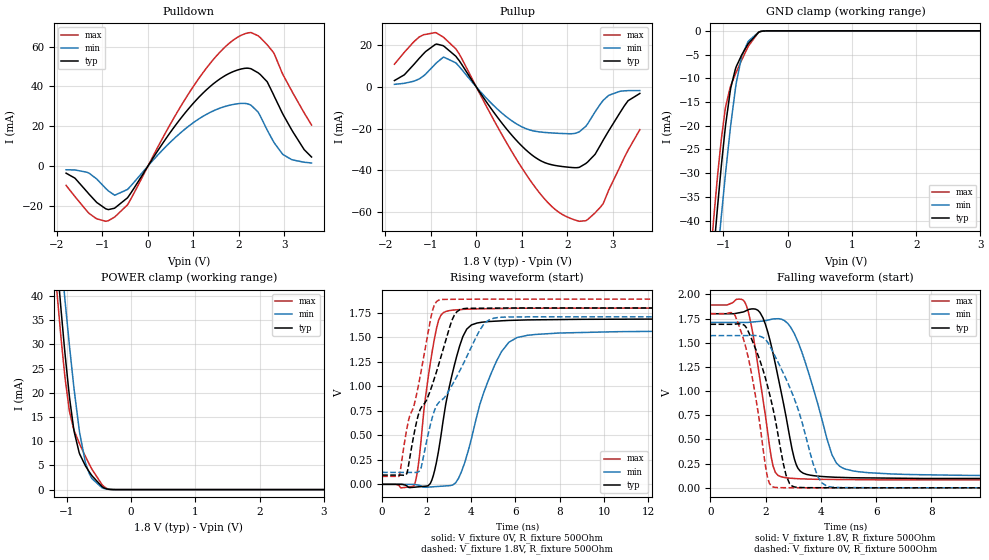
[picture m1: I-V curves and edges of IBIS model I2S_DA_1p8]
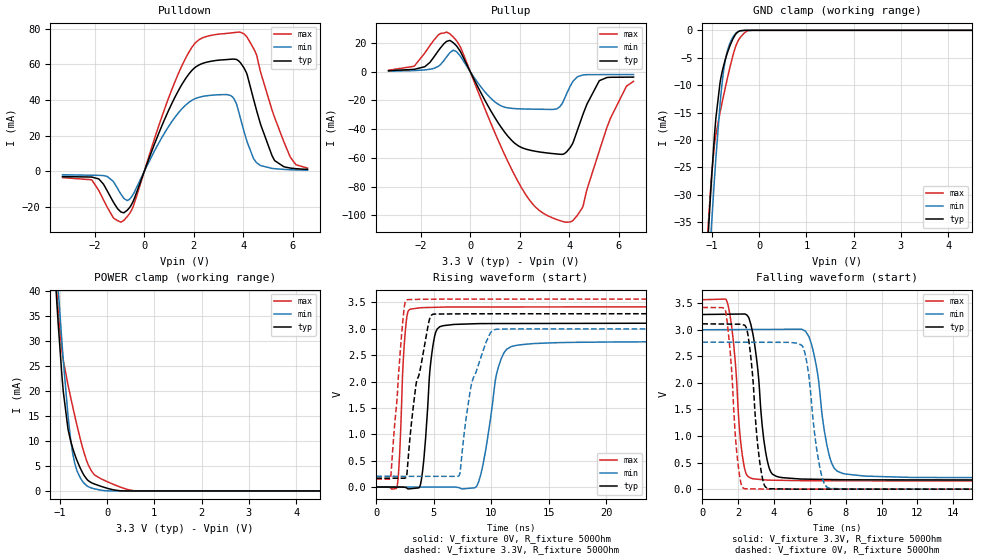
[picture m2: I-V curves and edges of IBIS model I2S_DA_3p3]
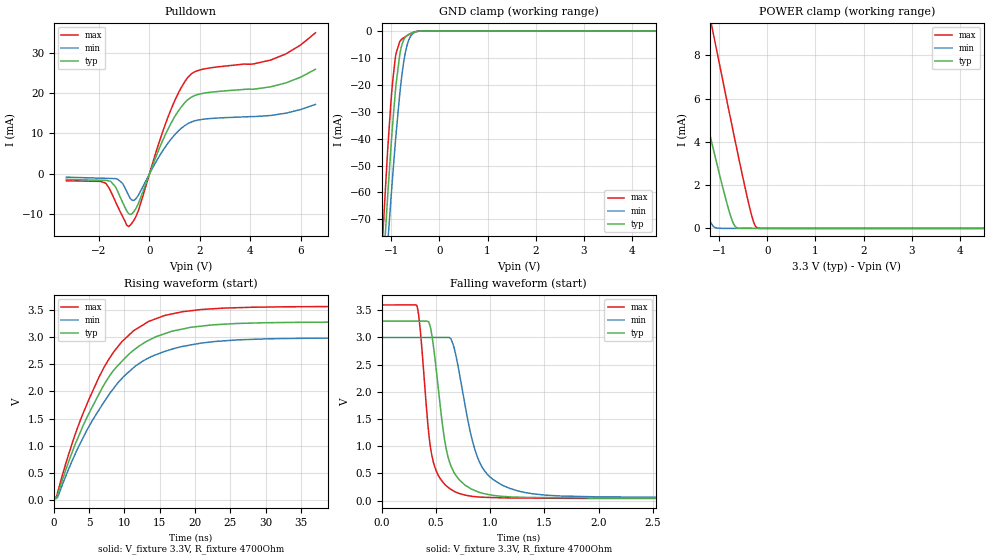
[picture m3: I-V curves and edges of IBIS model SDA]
| Texas Instruments Incorporated
| DS90UH928Q
| 5-85MHz 24-bit Color FPD-Link III to FPD-Link Deserializer with HDCP
| Marketing part#   Voltage Range   Package-type   Temperature
| DS90UH928QSQE   1.71V - 3.6V   48-Pin LLP   -40 to 105C
| DS90UH928QSQ   1.71V - 3.6V   48-Pin LLP   -40 to 105C
| DS90UH928QSQX   1.71V - 3.6V   48-Pin LLP   -40 to 105C
[IBIS Ver]   4.1
[File name]   ds90uh928q.ibs
[File Rev]   1.1
[Date]   08/10/2015
[Source]   Model built from SPICE simulations at:
   Texas Instruments Incorporated.
   WEBENCH DESIGN CENTER
   12500 TI Blvd
   Dallas, TX -75243
[Notes]   Rev 1.1: 08/10/2015
   - Diff pin mapping corrected.
   Rev 1.0: 02/13/2013
   - Initial version of the IBIS model
   - All models are generated in Spectre
   - ccomp is listed in numerical order, for PVT information,
   please check notes above ccomp keyword for each model
   - All non-monotonic warnings can be ignored as they were reviewed and
   considered minor.
   - Models with trailing xxxx_1p8 and xxxx_3p3 represent 1.8V and 3.3V
   power supply operation respectively.
[Disclaimer] This product is designed as an aid for customers of Texas Instruments.
   No warranties, either expressed or implied, with respect to this third
   party software (if any) or with respect to its fitness for any
   particular purpose is claimed by Texas Instruments or the author. The
   software (if any) is provided solely on an "as is" basis. The entire
   risk as to its quality and performance is with the customer
[Copyright]   (C)Copyright 2013 Texas Instruments Incorporated.
   All rights reserved.
[Component]   DS90UH928Q
[Manufacturer]  Texas Instruments, Inc.
[Package]   |48-pin LLP
|   typ   min   max
R_pkg   0   0   0
L_pkg   0   0   0
C_pkg   0   0   0
[Pin]   signal_name   model_name   R_pin   L_pin   C_pin
1   PDB   PDB
2   CAPI2S   NC
3   I2S_DB/GPIO_REG5   I2S_DA
4   SDA   SDA
5   SCL   SDA
6   VDDIO   POWER
7   I2S_DA/GPIO_REG6   I2S_DA
8   I2S_CLK/GPIO_REG8   I2S_DA
9   BISTTEN   OEN
10   I2S_WC/GPIO_REG7   I2S_DA
11   MCLK   I2S_DA
12   IDX   NC
13   GPIO1   I2S_DA
14   GPIO0   I2S_DA
15   TXOUT3+   LVDS_OUT
16   TXOUT3-   LVDS_OUT
17   TXCLKOUT+   LVDS_OUT
18   TXCLKOUT-   LVDS_OUT
19   TXOUT2+   LVDS_OUT
20   TXOUT2-   LVDS_OUT
21   TXOUT1+   LVDS_OUT
22   TXOUT1-   LVDS_OUT
23   TXOUT0+   LVDS_OUT
24   TXOUT0-   LVDS_OUT
25   CAPLV25   NC
26   MAPSEL   OEN
27   LOCK   I2S_DA
28   PASS   I2S_DA
29   CAPLV12   NC
30   OEN   OEN
31   VDD33_B   POWER
32   LFMODE   OEN
33   CAPL12   NC
34   RES0   NC
35   OSS_SEL   OEN
36   I2S_DD/GPIO3   I2S_DA
37   I2S_DC/GPIO2   I2S_DA
38   VDD33_A   POWER
39   RES1   NC
40   RIN+   RX_CML_RCV
41   RIN-   RX_CML_RCV
42   CMF   NC
43   BISTC/INTB_IN   OEN
44   CMLOUTP   RX_CML
45   CMLOUTN   RX_CML
46   CAPR12   NC
47   CAPP12   NC
48   MODE_SEL   NC
49   DAP   GND
[Package Model] LLP48DS90UH928QSQ
[Diff pin]  inv_pin  vdiff  tdelay_typ  tdelay_min  tdelay_max
17   18   NA   NA   NA   NA
15   16   NA   NA   NA   NA
19   20   NA   NA   NA   NA
21   22   NA   NA   NA   NA
23   24   NA   NA   NA   NA
40   41   0.2   NA   NA   NA
44   45   0.2   NA   NA   NA
|   Model Selectors
[Model Selector]  I2S_DA
I2S_DA_3p3   3.3V operation
I2S_DA_1p8   3.3V operation
[Model Selector]  OEN
OEN_3p3   3.3V operation
OEN_1p8   3.3V operation
[Define Package Model]  LLP48DS90UH928QSQ
[Manufacturer]  Texas Instruments
[OEM]  Texas Instruments
[Description]  None
[Number Of Pins]  49
[Pin Numbers]
|Pin Num   Terminal Name
1   | L1:1
2   | L2:2
3   | L3:3
4   | L4:4
5   | L5:5
6   | L6:6
7   | L7:7
8   | L8:8
9   | L9:9
10   | L10:10
11   | L11:11
12   | L12:12
13   | L13:13
14   | L14:14
15   | L15:15
16   | L16:16
17   | L17:17
18   | L18:18
19   | L19:19
20   | L20:20
21   | L21:21
22   | L22:22
23   | L23:23
24   | L24:24
25   | L25:25
26   | L26:26
27   | L27:27
28   | L28:28
29   | L29:29
30   | L30:30
31   | L31:31
32   | L32:32
33   | L33:33
34   | L34:34
35   | L35:35
36   | L36:36
37   | L37:37
38   | L38:38
39   | L39:39
40   | L40:40
41   | L41:41
42   | L42:42
43   | L43:43
44   | L44:44
45   | L45:45
46   | L46:46
47   | L47:47
48   | L48:48
49   | LDAP:49
[Model Data]
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[End Model Data]
[End Package Model]
| Models and submodels in the file (9): I2S_DA_1p8 (I/O), I2S_DA_3p3 (I/O), SDA (I/O_open_drain), RX_CML_RCV (Input), RX_CML (Output), PDB (Input), OEN_3p3 (Input), OEN_1p8 (Input), LVDS_OUT (Output)
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|   Model
[Model]   I2S_DA_1p8
Model_type   I/O
Polarity   Non-Inverting
Enable   Active-Low
Vinl = 0.63
Vinh = 1.17
Vmeas = 0.9
Vref = 0
Cref = 1pF
Rref = 1000000
|   typ   min   max
C_comp   1.5999pF   1.5084pF   1.9148pF
[Voltage Range]   1.8   1.71   1.89
[Temperature Range]   25   105   -40
[Pullup Reference]   1.8   1.71   1.89
[Pulldown Reference]   0   0   0
[Power Clamp Reference]   1.8   1.71   1.89
[GND Clamp Reference]   0   0   0
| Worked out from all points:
|   slope of the pulldown table from 0 to 0.27 V, typ, clamps not added: 28.2 ohm
|   slope of the pullup table from 0 to 0.27 V, typ, clamps not added: 31.1 ohm
|   GND clamp passes 1 mA (typ) near -0.50 V on its own axis
|   POWER clamp passes 1 mA (typ) near -0.48 V on its own axis
|   falling waveform, V_fixture 1.8V, R_fixture 500Ohm: 20-80 % time 720ps typ, 970ps min, 560ps max; typ from 1.8 V to 0.094 V
|   rising waveform, V_fixture 0V, R_fixture 500Ohm: 20-80 % time 877ps typ, 1.31ns min, 607ps max; typ from 0 V to 1.69 V
|   rising waveform, V_fixture 1.8V, R_fixture 500Ohm: 20-80 % time 1.48ns typ, 2ns min, 1.03ns max; typ from 0.094 V to 1.8 V
|   falling waveform, V_fixture 0V, R_fixture 500Ohm: 20-80 % time 835ps typ, 1.14ns min, 636ps max; typ from 1.69 V to 0 V
[Pulldown]
|   Voltage   I(typ)   I(min)   I(max)
-1.8V     -3.602mA   -1.89mA    -9.732mA
-1.13V    -18.2mA    -6.438mA   -26.49mA
-730.8mV  -21.14mA   -14.67mA   -25.6mA
-450mV    -15.96mA   -11.77mA   -19.49mA
457.2mV   15.8mA     11.21mA    19.63mA
1.105V    34.21mA    23.45mA    43.56mA
1.705V    45.5mA     29.98mA    59.98mA
2.196V    49.12mA    31.15mA    66.83mA
2.417V    46.85mA    27.15mA    65.43mA
2.617V    42.37mA    18.18mA    60.95mA
2.957V    26.38mA    5.999mA    46.3mA
3.595V    4.522mA    1.513mA    20.6mA
[GND Clamp]
|   Voltage   I(typ)   I(min)   I(max)
-1.8V     -162.6mA   -161mA     -166.7mA
-1.201V   -55.01mA   -64.35mA   -48.08mA
-1.152V   -46.98mA   -56.91mA   -39.96mA
-1.093V   -37.56mA   -48.01mA   -30.98mA
-1.039V   -29.54mA   -40.16mA   -23.8mA
-963mV    -19.69mA   -29.71mA   -15.92mA
-892.8mV  -12.73mA   -20.82mA   -11.89mA
-795.6mV  -7.443mA   -10.75mA   -8.613mA
-714.6mV  -5.105mA   -5.442mA   -6.162mA
-617.4mV  -2.827mA   -2.355mA   -3.43mA
-450mV    -299.1uA   -264.1uA   -281.1uA
3.595V    0A         0A         0A
[Pullup]
|   Voltage   I(typ)   I(min)   I(max)
-1.8V     3.07mA     1.252mA    10.93mA
-1.255V   13.76mA    3.863mA    24.05mA
-903.6mV  20.4mA     10.96mA    26.16mA
-714.6mV  19.65mA    14.35mA    23.79mA
-374.4mV  12.6mA     9.801mA    15.82mA
457.2mV   -14.35mA   -10.52mA   -18.8mA
1.094V    -30.36mA   -20.07mA   -42.03mA
1.667V    -37.47mA   -22.14mA   -57.64mA
2.25V     -38.72mA   -21.72mA   -64.53mA
2.785V    -25.75mA   -6.573mA   -56.24mA
3.335V    -6.631mA   -1.777mA   -30.42mA
3.595V    -3.131mA   -1.752mA   -20.54mA
[POWER Clamp]
|   Voltage   I(typ)   I(min)   I(max)
-1.8V     161.3mA    160.4mA    165mA
-1.157V   48.1mA     58.18mA    41.7mA
-1.087V   37.06mA    47.82mA    31.19mA
-1.033V   29.11mA    40.11mA    24.06mA
-957.6mV  19.26mA    29.82mA    16.3mA
-882mV    11.86mA    20.43mA    12.15mA
-795.6mV  7.282mA    11.52mA    9.335mA
-709.2mV  4.933mA    5.625mA    6.87mA
-606.6mV  2.86mA     2.271mA    4.196mA
-450mV    607.2uA    381.3uA    1.019mA
-266.4mV  7.62uA     8.999uA    8.268uA
3.595V    0A         0A         0A
[Ramp]
R_load = 500
|   typ   min   max
dV/dt_r   1.01367/8.76582e-10   0.941883/1.31022e-09   1.0806/6.06669e-10
dV/dt_f   1.02351/7.20399e-10   0.952642/9.69527e-10   1.08535/5.60273e-10
[Falling Waveform]
V_fixture = 1.8V
V_fixture_min = 1.71V
V_fixture_max = 1.89V
R_fixture = 500Ohm
C_fixture = 0F
|   Time   V(typ)   V(min)   V(max)
0s        1.8V       1.71V      1.89V
1.301ns   1.832V     1.71V      1.885V
1.791ns   1.814V     1.722V     1.127V
2.269ns   1.388V     1.746V     225.1mV
2.643ns   876.4mV    1.735V     109.2mV
3.038ns   301.6mV    1.595V     97.02mV
3.255ns   171.8mV    1.447V     93.41mV
4.404ns   111.4mV    341.2mV    87.05mV
5.171ns   104.5mV    174.8mV    85.19mV
30ns      94.14mV    122.3mV    81.06mV
[Rising Waveform]
V_fixture = 0V
V_fixture_min = 0V
V_fixture_max = 0V
R_fixture = 500Ohm
C_fixture = 0F
|   Time   V(typ)   V(min)   V(max)
0s        4.816uV    9.619uV    3.008uV
1.493ns   -28.51mV   -2.803mV   21.83mV
2.243ns   45.32mV    -25.87mV   1.338V
2.544ns   345mV      -21.27mV   1.674V
2.894ns   849.8mV    -15.93mV   1.766V
3.311ns   1.264V     14.84mV    1.78V
3.81ns    1.583V     289.4mV    1.788V
5.032ns   1.664V     1.196V     1.793V
6.083ns   1.675V     1.498V     1.797V
30ns      1.689V     1.57V      1.801V
[Rising Waveform]
V_fixture = 1.8V
V_fixture_min = 1.71V
V_fixture_max = 1.89V
R_fixture = 500Ohm
C_fixture = 0F
|   Time   V(typ)   V(min)   V(max)
0s        94.11mV    122.2mV    81.06mV
776.8ps   94.16mV    121.5mV    89.81mV
1.124ns   117.9mV    121.2mV    580.5mV
1.706ns   758.9mV    142.7mV    1.094V
2.269ns   1.022V     689.8mV    1.774V
2.544ns   1.22V      832.6mV    1.879V
3.361ns   1.759V     1.099V     1.888V
4.561ns   1.797V     1.628V     1.889V
5.171ns   1.798V     1.701V     1.889V
30ns      1.8V       1.71V      1.89V
[Falling Waveform]
|Gnd
V_fixture = 0V
V_fixture_min = 0V
V_fixture_max = 0V
R_fixture = 500Ohm
C_fixture = 0F
|   Time   V(typ)   V(min)   V(max)
0s        1.691V     1.574V     1.802V
990.8ps   1.696V     1.574V     1.71V
1.504ns   1.529V     1.576V     1.157V
2.041ns   1.083V     1.518V     145.5mV
2.269ns   814.3mV    1.402V     9.432mV
2.643ns   246mV      1.184V     1.524mV
2.867ns   42.58mV    1.042V     1.319mV
3.893ns   1.5mV      114.2mV    464.1uV
4.404ns   985.5uV    6.822mV    455.2uV
30ns      18.46uV    39.95uV    10.33uV
|   Model
[Model]   I2S_DA_3p3
Model_type   I/O
Polarity   Non-Inverting
Enable   Active-Low
Vinl = 0.8
Vinh = 2
Vmeas = 1.65
Vref = 0
Cref = 1pF
Rref = 1000000
|   typ   min   max
C_comp   1.5999pF   1.5084pF   1.9148pF
[Voltage Range]   3.3   3   3.6
[Temperature Range]   25   105   -40
[Pullup Reference]   3.3   3   3.6
[Pulldown Reference]   0   0   -0
[Power Clamp Reference]   3.3   3   3.6
[GND Clamp Reference]   0   -0   0
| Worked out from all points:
|   slope of the pulldown table from 0 to 0.495 V, typ, clamps not added: 27.2 ohm
|   slope of the pullup table from 0 to 0.495 V, typ, clamps not added: 29.4 ohm
|   GND clamp passes 1 mA (typ) near -0.52 V on its own axis
|   POWER clamp passes 1 mA (typ) near -0.15 V on its own axis
|   falling waveform, V_fixture 3.3V, R_fixture 500Ohm: 20-80 % time 547ps typ, 705ps min, 459ps max; typ from 3.29 V to 0.169 V
|   rising waveform, V_fixture 0V, R_fixture 500Ohm: 20-80 % time 631ps typ, 1.15ns min, 401ps max; typ from 0 V to 3.11 V
|   rising waveform, V_fixture 3.3V, R_fixture 500Ohm: 20-80 % time 1.31ns typ, 1.55ns min, 725ps max; typ from 0.168 V to 3.29 V
|   falling waveform, V_fixture 0V, R_fixture 500Ohm: 20-80 % time 458ps typ, 570ps min, 412ps max; typ from 3.11 V to 0 V
[Pulldown]
|   Voltage   I(typ)   I(min)   I(max)
-3.3V     -2.905mA   -1.903mA   -3.487mA
-1.845V   -4.191mA   -2.225mA   -10.53mA
-825mV    -23.24mA   -15.16mA   -27.48mA
-458.7mV  -17.06mA   -13.07mA   -20.03mA
838.2mV   29.71mA    21.98mA    35.7mA
1.818V    54.9mA     38.87mA    67.25mA
3.472V    62.85mA    42.63mA    77.57mA
3.828V    61.71mA    32.59mA    78.09mA
4.412V    40.42mA    7.131mA    68.97mA
5.254V    6.237mA    1.524mA    30.5mA
5.897V    1.863mA    934.9uA    7.885mA
6.59V     1.078mA    679uA      1.807mA
[GND Clamp]
|   Voltage   I(typ)   I(min)   I(max)
-3.3V     -460mA     -423.9mA   -501.5mA
-1.073V   -36.94mA   -45.07mA   -35.22mA
-1.063V   -35.41mA   -43.62mA   -33.84mA
-1.013V   -28.09mA   -36.56mA   -27.51mA
-1.003V   -26.71mA   -35.18mA   -26.38mA
-914.1mV  -16.06mA   -23.41mA   -19.06mA
-825mV    -9.505mA   -13.43mA   -14.97mA
-745.8mV  -6.327mA   -7.116mA   -11.73mA
-617.1mV  -2.836mA   -2.348mA   -6.773mA
-419.1mV  -144.9uA   -143.6uA   -1.548mA
-132mV    -33.32nA   -83.84nA   -493.6nA
6.59V     0A         0A         0A
[Pullup]
|   Voltage   I(typ)   I(min)   I(max)
-3.3V     733uA      422.9uA    1.047mA
-1.845V   3.487mA    1.261mA    12.89mA
-825mV    21.85mA    13.3mA     26.44mA
-379.5mV  13.39mA    10.25mA    16.46mA
1.68V     -48.01mA   -25.51mA   -68.38mA
2.64V     -55.46mA   -26.1mA    -94.48mA
3.491V    -57.32mA   -25.83mA   -103mA
3.887V    -55.85mA   -15.31mA   -104.9mA
4.531V    -30.54mA   -2.272mA   -94.57mA
5.204V    -6.337mA   -1.995mA   -55.33mA
5.669V    -3.846mA   -1.979mA   -32mA
6.59V     -3.726mA   -1.961mA   -6.65mA
[POWER Clamp]
|   Voltage   I(typ)   I(min)   I(max)
-3.3V     458.5mA    424mA      498.8mA
-1.082V   40.82mA    47.39mA    42.47mA
-1.053V   36.34mA    43.15mA    38.45mA
-1.033V   33.45mA    40.37mA    35.94mA
-924mV    19.77mA    25.99mA    26.02mA
-825mV    12.34mA    14.99mA    21.17mA
-735.9mV  8.878mA    8.069mA    17.26mA
-627mV    5.889mA    3.864mA    12.75mA
-389.4mV  1.994mA    814.3uA    5.052mA
-132mV    937.8uA    161.4uA    2.443mA
561mV     0A         0A         44.45uA
6.59V     0A         0A         0A
[Ramp]
R_load = 500
|   typ   min   max
dV/dt_r   1.86529/6.30855e-10   1.65454/1.14623e-09   2.05076/4.01389e-10
dV/dt_f   1.87026/5.43355e-10   1.67581/7.00491e-10   2.04655/4.58036e-10
[Falling Waveform]
V_fixture = 3.3V
V_fixture_min = 3V
V_fixture_max = 3.6V
R_fixture = 500Ohm
C_fixture = 0F
|   Time   V(typ)   V(min)   V(max)
0s        3.286V     2.999V     3.564V
1.413ns   3.292V     3.002V     3.492V
2.214ns   3.295V     3.003V     677.9mV
2.736ns   3.056V     3.004V     203.9mV
3.524ns   713.9mV    3.005V     173.4mV
4.134ns   240.4mV    3.006V     167.6mV
5.945ns   188mV      2.87V      157.9mV
7.071ns   181.7mV    650.4mV    157.4mV
7.806ns   177.7mV    298.9mV    157.3mV
30ns      169.2mV    206.1mV    153.4mV
[Rising Waveform]
V_fixture = 0V
V_fixture_min = 0V
V_fixture_max = 0V
R_fixture = 500Ohm
C_fixture = 0F
|   Time   V(typ)   V(min)   V(max)
0s        6.519uV    10.19uV    508.7nV
1.805ns   -114.1uV   2.453uV    4.229mV
2.427ns   -3.741mV   -213.9nV   2.689V
2.91ns    -32.89mV   -2.285uV   3.367V
3.914ns   130.3mV    -6.59uV    3.401V
4.781ns   2.454V     -10.31uV   3.406V
5.509ns   3.039V     -13.43uV   3.41V
8.796ns   3.098V     44.76mV    3.414V
11.71ns   3.1V       2.662V     3.414V
30ns      3.109V     2.758V     3.418V
[Rising Waveform]
V_fixture = 3.3V
V_fixture_min = 3V
V_fixture_max = 3.6V
R_fixture = 500Ohm
C_fixture = 0F
|   Time   V(typ)   V(min)   V(max)
0s        168.4mV    203.6mV    153mV
1.255ns   167.9mV    203.4mV    175.4mV
2.225ns   167.6mV    203.3mV    2.955V
2.605ns   190.7mV    203.3mV    3.545V
3.47ns    1.968V     203.2mV    3.558V
4.902ns   3.275V     203.1mV    3.562V
7.209ns   3.283V     222.6mV    3.563V
8.285ns   3.285V     1.973V     3.563V
10.13ns   3.285V     2.968V     3.563V
30ns      3.286V     2.999V     3.564V
[Falling Waveform]
|Gnd
V_fixture = 0V
V_fixture_min = 0V
V_fixture_max = 0V
R_fixture = 500Ohm
C_fixture = 0F
|   Time   V(typ)   V(min)   V(max)
0s        3.111V     2.765V     3.418V
1.294ns   3.106V     2.765V     3.354V
1.94ns    3.104V     2.764V     629.8mV
2.345ns   3.087V     2.764V     9.947mV
3.22ns    471.8mV    2.763V     3.007mV
3.633ns   14.37mV    2.763V     552.1uV
5.605ns   742uV      2.68V      511.4uV
6.551ns   714uV      419.4mV    491.9uV
7.113ns   697.3uV    14.14mV    480.3uV
30ns      18.91uV    50.05uV    8.534uV
|   Model
[Model]   SDA
Model_type   I/O_open_drain
Polarity   Non-Inverting
Enable   Active-Low
Vinl = 0.8
Vinh = 2
Vmeas = 1.65
Vref = 3.3
Cref = 1pF
Rref = 4700
|   typ   min   max
C_comp   0.9710pF   0.8915pF   1.0265pF
[Voltage Range]   3.3   3   3.6
[Temperature Range]   25   105   -40
[Pullup Reference]   3.3   3   3.6
[Pulldown Reference]   0   0   0
[Power Clamp Reference]   3.3   3   3.6
[GND Clamp Reference]   0   0   0
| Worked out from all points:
|   slope of the pulldown table from 0 to 0.495 V, typ, clamps not added: 63.4 ohm
|   GND clamp passes 1 mA (typ) near -0.62 V on its own axis
|   POWER clamp passes 1 mA (typ) near -0.82 V on its own axis
|   falling waveform, V_fixture 3.3V, R_fixture 4700Ohm: 20-80 % time 140ps typ, 209ps min, 105ps max; typ from 3.3 V to 0.04 V
|   rising waveform, V_fixture 3.3V, R_fixture 4700Ohm: 20-80 % time 8.24ns typ, 8.7ns min, 7.55ns max; typ from 0.04 V to 3.3 V
[Pulldown]
|   Voltage   I(typ)   I(min)   I(max)
-3.3V     -1.332mA   -798uA     -1.685mA
-1.756V   -1.589mA   -1.077mA   -2.211mA
-1.528V   -1.894mA   -1.115mA   -4.392mA
-1.27V    -4.15mA    -1.258mA   -7.916mA
-815.1mV  -9.859mA   -5.451mA   -12.98mA
-528mV    -8.462mA   -6.067mA   -10.42mA
699.6mV   10.6mA     7.313mA    13.44mA
1.115V    15.26mA    10.42mA    19.59mA
1.531V    18.39mA    12.45mA    23.91mA
2.165V    19.97mA    13.54mA    25.95mA
4.818V    21.55mA    14.45mA    28.17mA
6.59V     25.88mA    17.2mA     34.89mA
[GND Clamp]
|   Voltage   I(typ)   I(min)   I(max)
-3.3V     -766.2mA   -698.7mA   -829.3mA
-1.191V   -94.72mA   -109.2mA   -79.97mA
-1.082V   -63.01mA   -80.79mA   -45.96mA
-1.073V   -60.26mA   -78.27mA   -43.12mA
-1.013V   -44.43mA   -63.54mA   -27.47mA
-973.5mV  -34.7mA    -54.11mA   -18.78mA
-904.2mV  -20.1mA    -38.66mA   -8.432mA
-825mV    -8.769mA   -23.36mA   -3.891mA
-716.1mV  -2.461mA   -8.696mA   -2.188mA
-587.4mV  -754.8uA   -1.63mA    -911.4uA
-270.6mV  -546.8nA   -2.071uA   -78.56nA
6.59V     0A         0A         0A
[POWER Clamp]
|   Voltage   I(typ)   I(min)   I(max)
-3.3V     24.92mA    17.48mA    33.59mA
-2.478V   16.78mA    10.48mA    24.23mA
-2.28V    14.83mA    8.815mA    21.98mA
-1.795V   10.08mA    4.789mA    16.5mA
-1.597V   8.164mA    3.193mA    14.28mA
-1.31V    5.412mA    1.035mA    11.07mA
-1.132V   3.738mA    116.5uA    9.086mA
-1.092V   3.371mA    45.51uA    8.648mA
-686.4mV  147.5uA    469.2nA    4.218mA
-359.7mV  496.7nA    234nA      882.7uA
-211.2mV  371.6nA    171.2nA    24.78uA
6.59V     0A         0A         0A
[Ramp]
R_load = 4700
|   typ   min   max
dV/dt_r   1.95464/8.2302e-09   1.76747/8.70017e-09   2.13685/7.55509e-09
dV/dt_f   1.95461/1.39661e-10   1.76747/2.0862e-10   2.13685/1.04609e-10
[Falling Waveform]
V_fixture = 3.3V
V_fixture_min = 3V
V_fixture_max = 3.6V
R_fixture = 4700Ohm
C_fixture = 0F
|   Time   V(typ)   V(min)   V(max)
0s        3.298V     2.998V     3.597V
327.3ps   3.298V     2.999V     3.56V
447.4ps   3.196V     2.999V     1.001V
578.7ps   1.129V     2.999V     303.6mV
657.7ps   551.7mV    2.874V     183.6mV
836.7ps   203.6mV    1.092V     77.21mV
947ps     125.8mV    548.4mV    60.88mV
1.186ns   68.6mV     220.2mV    48.71mV
1.706ns   52.41mV    82.26mV    41.25mV
500ns     40.41mV    52.32mV    35.37mV
[Rising Waveform]
V_fixture = 3.3V
V_fixture_min = 3V
V_fixture_max = 3.6V
R_fixture = 4700Ohm
C_fixture = 0F
|   Time   V(typ)   V(min)   V(max)
0s        40.35mV    52.32mV    35.37mV
300.3ps   33.73mV    52.8mV     21.07mV
525ps     88.06mV    43.31mV    128.7mV
2.644ns   894.9mV    734.9mV    1.062V
4.894ns   1.573V     1.334V     1.83V
7.061ns   2.113V     1.795V     2.434V
9.643ns   2.556V     2.241V     2.92V
14.52ns   3.014V     2.681V     3.345V
24.09ns   3.241V     2.934V     3.538V
500ns     3.298V     2.998V     3.597V
